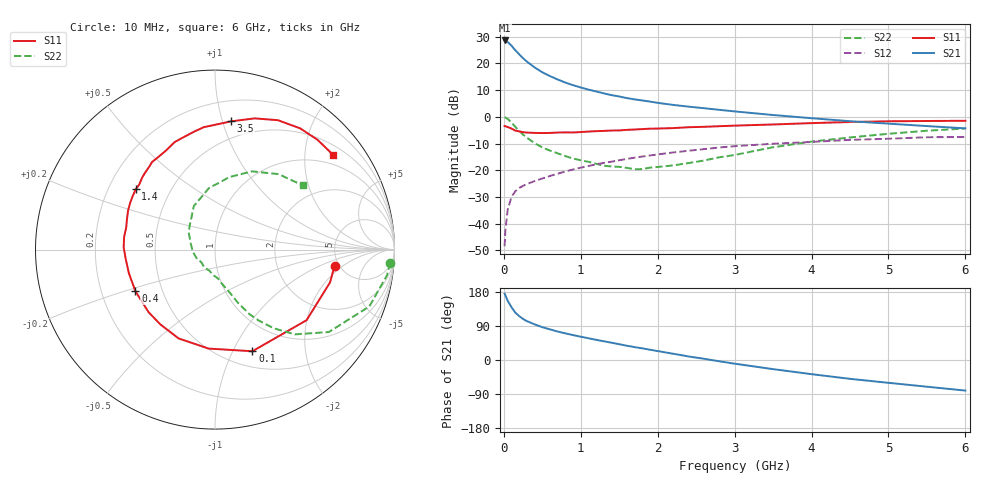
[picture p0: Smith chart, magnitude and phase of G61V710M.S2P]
! SIEMENS Small Signal Semiconductors
! BFG193
! Si NPN RF Bipolar Junction Transistor in SOT223
! VCE = 1.75 V  IC = 10 mA
! Common Emitter S-Parameters:  August  1996
# GHz  S  MA  R  50
!  f  S11  S21  S12  S22
! GHz  MAG  ANG  MAG  ANG  MAG  ANG  MAG  ANG
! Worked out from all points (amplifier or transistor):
!   36 points, 10 MHz to 6 GHz, reference 50 ohm
!   highest |S21| = 28.6 dB at 10 MHz (marker M1)
!   |S21| within 3 dB of that: start of sweep to 129.8 MHz
!   unconditionally stable (mu >= 1): 852.1 MHz to 2.727 GHz
!   at 250 MHz: K = 0.54, MSG = 23.9 dB, |S12| = -25.8 dB
!   at 1.4 GHz: K = 1.07, MAG = 10.8 dB, |S12| = -16.8 dB
!   at 6 GHz: K = 0.92, MSG = 1.6 dB, |S12| = -7.5 dB
!   S11 on the Smith chart (normalised r, x): 10 MHz: 4.57, -1.52; 100 MHz: 0.67, -1.20; 400 MHz: 0.35, -0.22; 1.4 GHz: 0.32, +0.31; 3.5 GHz: 0.36, +1.07; 6 GHz: 0.72, +2.66
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0.01  0.6722 -7.8  26.9 175.0  0.0038 90.5  0.9789 -4.3
0.02  0.6666 -15.9  26.7 170.8  0.0076 84.1  0.969 -8.5
0.05  0.6442 -37.6  25.15 156.3  0.0182 72.3  0.9166 -20.2
0.1  0.6035 -69.8  21.47 139.1  0.032 62.6  0.7831 -35.9
0.15  0.5526 -93.7  17.57 124.9  0.0405 54.0  0.649 -46.7
0.2  0.5349 -112.3  14.79 115.7  0.0467 51.0  0.548 -53.2
0.25  0.516 -126.2  12.51 108.2  0.0511 48.4  0.4634 -58.4
0.3  0.5085 -136.7  10.79 102.6  0.0552 48.0  0.4078 -61.9
0.4  0.5004 -152.4  8.42 94.0  0.0628 47.4  0.3219 -66.7
0.5  0.4976 -164.7  6.827 86.6  0.0702 47.5  0.2679 -69.9
0.6  0.5001 -173.9  5.787 80.7  0.0783 48.2  0.2336 -73.0
0.7  0.5091 178.5  5.003 75.2  0.0863 48.4  0.2075 -76.5
0.9  0.51 165.9  3.917 65.7  0.1036 47.7  0.1658 -82.9
1.1  0.5307 155.9  3.234 57.4  0.1203 46.7  0.1441 -93.4
1.4  0.5549 142.7  2.551 45.6  0.145 42.9  0.118 -111.4
1.7  0.5795 132.1  2.123 34.0  0.1721 38.8  0.1046 -134.3
2.2  0.6158 116.3  1.674 16.6  0.2155 29.2  0.1234 -174.2
2.8  0.6682 99.8  1.354 -3.4  0.2671 16.9  0.1749 146.9
3.5  0.72 82.9  1.082 -24.1  0.314 0.5  0.2698 115.9
4.5  0.8015 64.1  0.829 -49.7  0.3706 -19.2  0.4115 78.8
5.5  0.8368 47.0  0.672 -70.5  0.4156 -42.5  0.5497 49.9
6  0.8436 38.9  0.609 -80.7  0.4193 -55.9  0.6059 36.2
